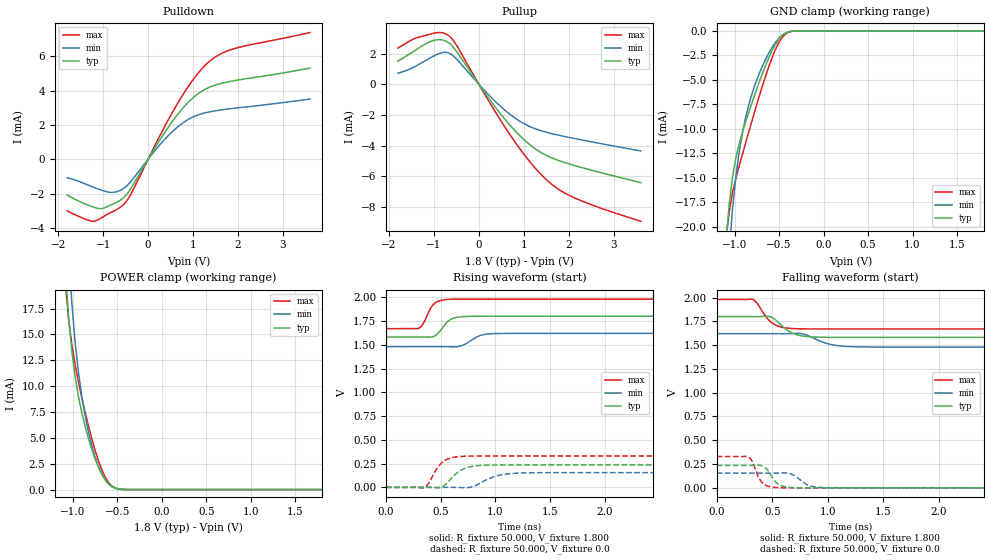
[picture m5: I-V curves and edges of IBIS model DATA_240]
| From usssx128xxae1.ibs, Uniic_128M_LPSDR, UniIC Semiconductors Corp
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|   Model DATA_240
[Model] DATA_240
Model_type I/O
Polarity   Inverting
Enable   Active-High
Vinl =  0.0V
Vinh =  1.800V
Vmeas =  0.900V
Vref =  0.900V
C_comp   1.060pF   1.050pF   1.070pF
[Model Spec]
Vinh   1.800V   1.400V   2.100V
Vinl   0.0V   -0.300V   0.400V
Vmeas   0.900V   0.810V   0.990V
Vref   0.900V   0.810V   0.990V
[Temperature Range]   25.000   0.125k   -40.000
[Voltage Range]   1.800V   1.620V   1.980V
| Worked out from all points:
|   slope of the pulldown table from 0 to 0.27 V, typ, clamps not added: 232 ohm
|   slope of the pullup table from 0 to 0.27 V, typ, clamps not added: 241 ohm
|   GND clamp passes 1 mA (typ) near -0.51 V on its own axis
|   POWER clamp passes 1 mA (typ) near -0.64 V on its own axis
|   rising waveform, R_fixture 50.000, V_fixture 1.800: 20-80 % time 98.2ps typ, 125ps min, 83.3ps max; typ from 1.58 V to 1.8 V
|   rising waveform, R_fixture 50.000, V_fixture 0.0: 20-80 % time 141ps typ, 183ps min, 115ps max; typ from 0 V to 0.236 V
|   falling waveform, R_fixture 50.000, V_fixture 1.800: 20-80 % time 147ps typ, 186ps min, 124ps max; typ from 1.8 V to 1.58 V
|   falling waveform, R_fixture 50.000, V_fixture 0.0: 20-80 % time 89.4ps typ, 113ps min, 75.9ps max; typ from 0.236 V to 0 V
[Pulldown]
|Voltage   I(typ)   I(min)   I(max)
-1.8V     -2.092mA   -1.078mA   -3.001mA
-1.195V   -2.805mA   -1.65mA    -3.61mA
-1.03V    -2.876mA   -1.808mA   -3.397mA
-810mV    -2.64mA    -1.934mA   -3.075mA
-535mV    -2.211mA   -1.679mA   -2.605mA
-370mV    -1.644mA   -1.25mA    -1.967mA
235mV     1.018mA    761.4uA    1.236mA
675mV     2.667mA    1.919mA    3.334mA
1.06V     3.714mA    2.532mA    4.839mA
1.445V    4.272mA    2.798mA    5.864mA
1.995V    4.61mA     2.992mA    6.494mA
3.6V      5.309mA    3.508mA    7.374mA
[Pullup]
|Voltage   I(typ)   I(min)   I(max)
-1.8V     1.525mA    731uA      2.374mA
-1.405V   2.25mA     1.195mA    3.022mA
-1.075V   2.802mA    1.745mA    3.29mA
-855mV    2.917mA    2.043mA    3.382mA
-690mV    2.751mA    2.072mA    3.222mA
-525mV    2.257mA    1.735mA    2.675mA
190mV     -796uA     -604.5uA   -956uA
630mV     -2.463mA   -1.818mA   -3.026mA
1.07V     -3.794mA   -2.674mA   -4.832mA
1.455V    -4.575mA   -3.092mA   -6.104mA
2.115V    -5.296mA   -3.533mA   -7.406mA
3.6V      -6.422mA   -4.353mA   -8.949mA
[GND_clamp]
|Voltage   I(typ)   I(min)   I(max)
-1.8V     -271.7mA   -304.3mA   -257.9mA
-1.097V   -21.71mA   -28.04mA   -21.32mA
-1.06V    -17.73mA   -22.52mA   -18.46mA
-1.023V   -14.97mA   -18.24mA   -16.55mA
-986mV    -13.03mA   -14.97mA   -15.09mA
-912mV    -10.37mA   -10.44mA   -12.62mA
-801mV    -7.262mA   -6.333mA   -9.099mA
-690mV    -4.437mA   -3.666mA   -5.721mA
-579mV    -2.043mA   -1.694mA   -2.765mA
-431mV    -248.4uA   -247.4uA   -345.1uA
-283mV    -5.293uA   -10.2uA    -5.65uA
1.8V      0A         0A         0A
[POWER_clamp]
|Voltage   I(typ)   I(min)   I(max)
-1.8V     340.2mA    394mA      317.1mA
-1.086V   21.52mA    29.62mA    20.16mA
-1.049V   16.79mA    23.07mA    16.54mA
-1.012V   13.42mA    18.08mA    14.02mA
-975mV    10.94mA    14.29mA    12.08mA
-938mV    9.034mA    11.39mA    10.43mA
-901mV    7.488mA    9.092mA    8.933mA
-827mV    5.01mA     5.66mA     6.217mA
-716mV    2.228mA    2.327mA    2.865mA
-568mV    301.3uA    355.6uA    397.2uA
-420mV    7.103uA    18.41uA    6.039uA
1.8V      0A         0A         0A
[Ramp]
| variable   typ   min   max
dV/dt_r   0.142/0.141n   93.003m/0.184n   0.198/0.115n
dV/dt_f   0.131/0.148n   84.408m/0.186n   0.186/0.124n
R_load = 50.000
[Rising Waveform]
R_fixture= 50.000
V_fixture= 1.800
V_fixture_min= 1.620
V_fixture_max= 1.980
|time   V(typ)   V(min)   V(max)
0s        1.581V     1.479V     1.67V
304ps     1.581V     1.479V     1.676V
343ps     1.582V     1.479V     1.725V
407ps     1.58V      1.479V     1.881V
440ps     1.589V     1.479V     1.93V
606ps     1.774V     1.478V     1.978V
700ps     1.796V     1.494V     1.98V
867ps     1.8V       1.599V     1.98V
1.02ns    1.8V       1.618V     1.98V
10ns      1.8V       1.62V      1.98V
[Rising Waveform]
R_fixture= 50.000
V_fixture= 0.0
V_fixture_min= 0.0
V_fixture_max= 0.0
|time   V(typ)   V(min)   V(max)
0s        16.46nV    104nV      27.83nV
350ps     572.4uV    30.22uV    -3.054mV
384ps     635.3uV    25.76uV    32.17mV
462ps     -3.908mV   4.51uV     188.9mV
524ps     11.24mV    320.4uV    270.6mV
648ps     149.9mV    -614.8uV   321.6mV
740ps     207.2mV    -3.302mV   328.2mV
1.021ns   235.8mV    123.3mV    330.1mV
1.301ns   236.5mV    153.1mV    330.1mV
10ns      236.4mV    155mV      330.1mV
[Falling Waveform]
R_fixture= 50.000
V_fixture= 1.800
V_fixture_min= 1.620
V_fixture_max= 1.980
|time   V(typ)   V(min)   V(max)
0s        1.8V       1.62V      1.98V
325ps     1.799V     1.62V      1.979V
362ps     1.799V     1.62V      1.942V
454ps     1.803V     1.62V      1.784V
507ps     1.784V     1.62V      1.726V
629ps     1.662V     1.62V      1.679V
724ps     1.608V     1.623V     1.672V
1.043ns   1.581V     1.503V     1.67V
1.283ns   1.581V     1.481V     1.67V
10ns      1.581V     1.479V     1.67V
[Falling Waveform]
R_fixture= 50.000
V_fixture= 0.0
V_fixture_min= 0.0
V_fixture_max= 0.0
|time   V(typ)   V(min)   V(max)
0s        236.4mV    155mV      330.1mV
284ps     236.3mV    155mV      325mV
316ps     236.2mV    155mV      286.5mV
378ps     238.1mV    155mV      110.1mV
413ps     230.3mV    155mV      51.06mV
578ps     24.55mV    156.6mV    1.38mV
681ps     3.19mV     139.4mV    158.5uV
853ps     137.4uV    16.61mV    5.016uV
1.043ns   6.33uV     783.4uV    178.6nV
10ns      19.27nV    106.4nV    30.65nV
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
